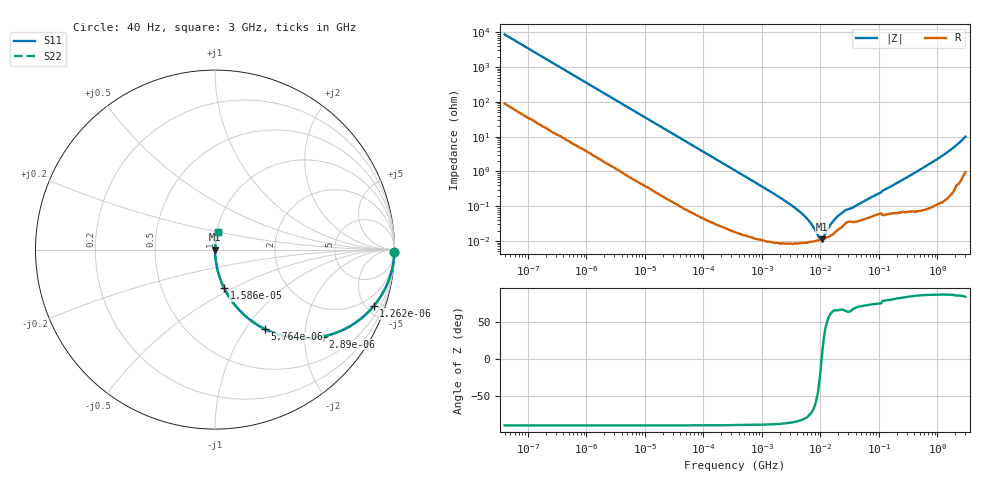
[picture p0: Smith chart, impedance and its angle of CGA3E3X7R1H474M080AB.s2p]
! S-parameter Generated by TDK Corporation
! Copyright(C) 2015 TDK Corporation.
! All Rights Reserved.
! TDK P/N: CGA3E3X7R1H474M080AB (Multilayer Ceramic Chip Capacitors)
! Property: C=470nF
! Size(LxWxT): 1.6x0.8x0.8mm, 0.063x0.031x0.031inches
! Model Type: s2p (Touchstone File Format Version 1.0)
! Frequency: DC=Yes Start=0.00004MHz Stop=3000MHz 396points Log-sweep
! Note: This model was converted from impedance.
! Model Generated on Jun. 23, 2015
! Hash(MD5):
! Port Assignments:
!  1 ---| |--- 2
! Applicable Conditions:
!  Temperature = 25 degC
!  DC Bias Voltage = 0 V
!  Small Signal Operation
! Terms and conditions regarding TDK Simulation Models
! (1)This simulation model is being provided solely for informational purposes. Please refer to the specifications of the products in terms of detailed characteristics of such products.
! (2)In no event shall TDK Corporation of any of its subsidiaries be liable for any loss or damage arising, directly or indirectly,
!  From any information contained in this simulation model, including, but not limited to loss or damages arising from any inaccuracies, omissions or errors in connection with such information.
! (3)Any and all copyrights on this simulation model are owned by TDK Corporation.
!  Duplication or redistribution of this simulation model without prior written permission from TDK Corporation is prohibited.
! (4)This simulation model is subject to any modification or change without any prior notice.
! (5)Neither TDK Corporation nor any of its subsidiaries shall make any warranty, express or implied,
!  Including but not limited to the correctness, implied warranties of merchantability and fitness for a particular purpose with respect to this simulation models.
! (6)The use of this simulation model shall be deemed to have consented to the terms and conditions hereof.
# MHz S MA R 50
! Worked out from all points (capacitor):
!   395 points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, 40 Hz to 3 GHz, reference 50 ohm
!   read as one part in series: C = 458 nF near 41.88 Hz
!   lowest |Z| = 11.1 mohm at 10.44 MHz (marker M1)
!   series resonance near 10.43 MHz, so ESL is about 510 pH
!   S11 on the Smith chart (normalised r, x): 40 Hz: open; 1.262 kHz: 1.06, -5.61; 2.89 kHz: 1.03, -2.46; 5.764 kHz: 1.01, -1.24; 15.86 kHz: 1.00, -0.45; 3 GHz: 1.02, +0.20
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4e-05  0.9998 -0.7  0.01154 88.7  0.01154 88.7  0.9998 -0.7
0.0002520917  0.9967 -4.1  0.07168 85.3  0.07168 85.3  0.9967 -4.1
0.000834128  0.9709 -13.3  0.2294 76.1  0.2294 76.1  0.9709 -13.3
0.001262176  0.9387 -19.6  0.3348 69.8  0.3348 69.8  0.9387 -19.6
0.002889976  0.7722 -38.8  0.6271 50.5  0.6271 50.5  0.7722 -38.8
0.005763764  0.5247 -57.8  0.8459 31.6  0.8459 31.6  0.5247 -57.8
0.009132315  0.3646 -68.0  0.9273 21.4  0.9273 21.4  0.3646 -68.0
0.01586465  0.2213 -76.6  0.9729 12.8  0.9729 12.8  0.2213 -76.6
0.01739424  0.2029 -77.7  0.9771 11.7  0.9771 11.7  0.2029 -77.7
0.05755453  0.06339 -85.7  0.9973 3.6  0.9973 3.6  0.06339 -85.7
0.3464102  0.0107 -88.4  0.9998 0.6  0.9998 0.6  0.0107 -88.4
3.154924  0.001082 -85.5  0.9999 0.1  0.9999 0.1  0.001082 -85.5
5.234209  0.0005426 -80.4  0.9999 0.0  0.9999 0.0  0.0005426 -80.4
7.22376  0.0002838 -70.3  0.9999 0.0  0.9999 0.0  0.0002838 -70.3
9.521122  0.0001249 -31.7  0.9999 0.0  0.9999 0.0  0.0001249 -31.7
10.4391  0.0001111 0.3  0.9999 -0.0  0.9999 -0.0  0.0001111 0.3
15.79611  0.000342 63.8  0.9998 -0.0  0.9998 -0.0  0.000342 63.8
23.90217  0.0006737 67.1  0.9997 -0.0  0.9997 -0.0  0.0006737 67.1
150.6385  0.003525 79.9  0.9994 -0.2  0.9994 -0.2  0.003525 79.9
1251.294  0.02929 85.7  0.9982 -1.7  0.9982 -1.7  0.02929 85.7
2173.747  0.05864 82.7  0.9942 -3.4  0.9942 -3.4  0.05864 82.7
3000  0.09893 78.9  0.9857 -5.7  0.9857 -5.7  0.09893 78.9
